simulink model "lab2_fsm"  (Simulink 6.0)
settings: Solver=ode45  StartTime=0.0  StopTime=32*33  RelTol=1e-3
undefined symbols (not defined in the file or in its folder): netlist
libraries: xbsIndex_r3 x8

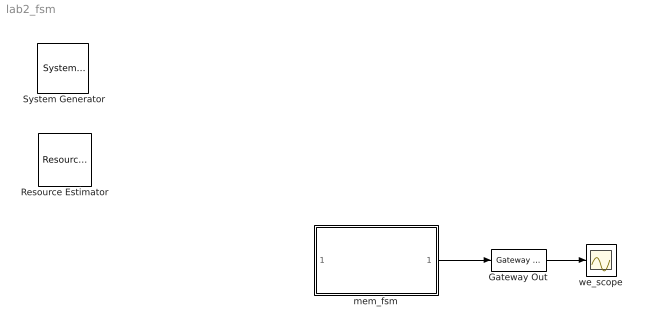
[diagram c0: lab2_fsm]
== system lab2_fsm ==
  " System Generator" : xbsIndex_r3/ System Generator  Tag=genX  xilinxfamily=Virtex2  part=xc2v1000  speed=-4  package=fg456  synthesis_tool=XST  directory=./netlist  testbench=off  simulink_period=1/2  sysclk_period=10  incr_netlist=off  trim_vbits=Everywhere in SubSystem  dbl_ovrd=According to Block Masks  core_generation=According to Block Masks  run_coregen=off  deprecated_control=off  eval_field=0
  Gateway Out : xbsIndex_r3/Gateway Out  output_type=Double  nbits=8  bin_pt=6  arith_type=Boolean  quantization=Truncate  overflow=Wrap  hdl_port=on  timing_constraint=None  locs_specified=off  LOCs={}  needs_fixed_name=off  show_param=off
  Resource Estimator : xbsIndex_r3/Resource Estimator  Tag=resEstTag  xl_estimator_area=[0 0 0 0 0 0 0]  xl_use_estimator_area=off  simulink_period=1/2  mrp_directory=./netlist
  mem_fsm : Subsystem
  we_scope : Scope
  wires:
  Gateway Out/1 -> we_scope/1
  mem_fsm/1(fsm_we_out) -> Gateway Out/1

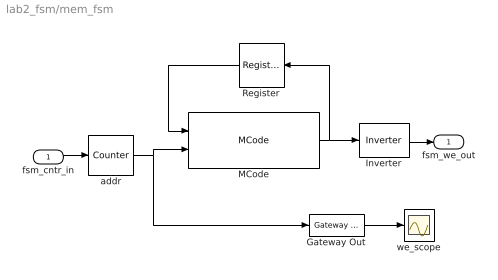
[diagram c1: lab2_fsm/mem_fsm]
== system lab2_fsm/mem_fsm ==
  fsm_cntr_in : Inport  Port=1  LatchInput=off
  Gateway Out : xbsIndex_r3/Gateway Out  output_type=Double  nbits=8  bin_pt=6  arith_type=Boolean  quantization=Truncate  overflow=Wrap  hdl_port=on  timing_constraint=None  locs_specified=off  LOCs={}  needs_fixed_name=off  show_param=off
  Inverter : xbsIndex_r3/Inverter  latency=0  explicit_period=off  period=1  en=off  dbl_ovrd=off  show_param=off
  MCode : xbsIndex_r3/MCode  mfname=lab2_fsm  defparams={}  suppress_output=off  hide_port_list={}  explicit_period=on  period=1  dbl_ovrd=off  show_param=off
  Register : xbsIndex_r3/Register  Orientation=left  init=0  reg_only_valid=off  explicit_period=on  period=1  rst=off  en=off  out_en=off  dbl_ovrd=off  show_param=off
  addr : xbsIndex_r3/Counter  Priority=5  cnt_type=Count Limited  n_bits=6  bin_pt=0  arith_type=Unsigned  start_count=0  cnt_to=32  cnt_by_val=1  operation=Up  explicit_period=off  period=1  load_pin=off  rst=off  en=on  dbl_ovrd=off  show_param=off  use_rpm=on  gen_core=on
  we_scope : Scope
  fsm_we_out : Outport
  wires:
  MCode/1 -> Register/1, Inverter/1
  Register/1 -> MCode/1
  addr/1 -> MCode/2, Gateway Out/1
  Inverter/1 -> fsm_we_out/1
  fsm_cntr_in/1 -> addr/1
  Gateway Out/1 -> we_scope/1
